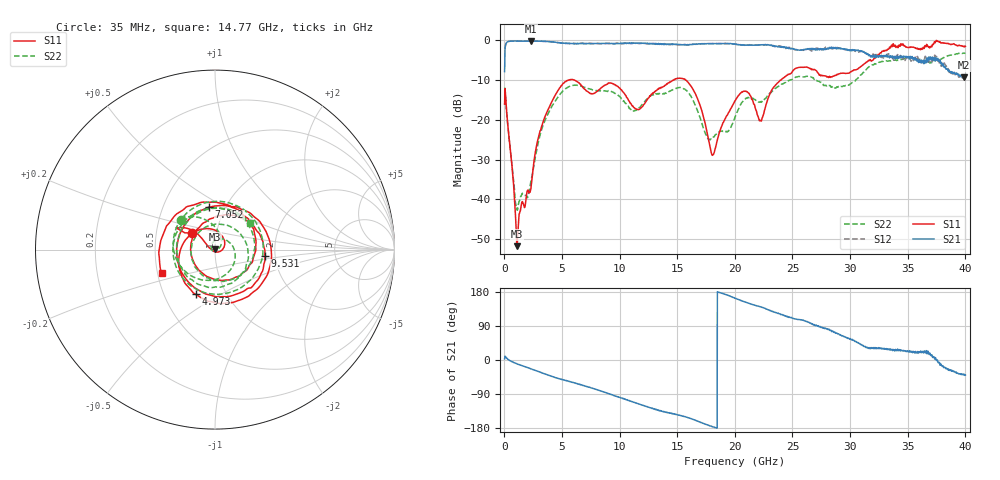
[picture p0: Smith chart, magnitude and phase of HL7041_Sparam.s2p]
! Created Wed Mar 30 16:31:27 2022
# ghz S ri R 50
! 2 Port Network Data from SP1.SP block
! freq  reS11  imS11  reS21  imS21  reS12  imS12  reS22  imS22
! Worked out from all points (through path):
!   2000 points, 35 MHz to 40 GHz, reference 50 ohm
!   highest |S21| = -0.13 dB at 2.354 GHz (marker M1); lowest = -9.3 dB at 39.86 GHz (marker M2)
!   group delay of S21, straight-line fit = 27.5 ps
!   lowest |S11| = -51.8 dB at 1.095 GHz (marker M3), VSWR 1.01, Z = 49.8 + j0.173 ohm
!   |S11| at or under -10 dB: start of sweep to 5.543 GHz; 6.107 GHz to 14.67 GHz (8.559 GHz wide, 82.4 % of centre); 15.75 GHz to 23.95 GHz (8.199 GHz wide, 41.3 % of centre)
!   |S22| runs from -42.7 to -3.2 dB; largest |S21 - S12| = 0.4
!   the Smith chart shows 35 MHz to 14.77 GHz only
!   S11 on the Smith chart (normalised r, x): 35 MHz: 0.76, +0.14; 4.973 GHz: 0.72, -0.39; 7.052 GHz: 0.84, +0.42; 9.531 GHz: 1.76, -0.14; 14.77 GHz: 0.53, -0.15
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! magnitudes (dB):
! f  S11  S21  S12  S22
! 35 MHz  -16.0  -7.8  -1.9  -12.1
! 1.095 GHz  -51.8  -0.1  -0.1  -42.2
! 2.354 GHz  -36.3  -0.1  -0.1  -35.0
! 3.214 GHz  -22.0  -0.2  -0.2  -22.7
! 4.973 GHz  -11.3  -0.7  -0.7  -13.1
! 6.712 GHz  -11.4  -0.8  -0.7  -11.6
! 7.052 GHz  -12.4  -0.8  -0.8  -11.9
! 9.531 GHz  -11.1  -0.8  -0.8  -13.2
! 11.57 GHz  -17.4  -0.7  -0.7  -17.3
! 13.37 GHz  -12.3  -0.8  -0.9  -13.5
! 14.77 GHz  -9.8  -1.0  -0.9  -12.2
! 16.47 GHz  -12.8  -1.0  -0.9  -15.6
! 18.07 GHz  -28.9  -0.8  -0.8  -24.7
! 20.03 GHz  -15.2  -0.9  -0.9  -19.2
! 21.09 GHz  -12.9  -1.2  -1.1  -14.4
! 22.25 GHz  -20.2  -1.1  -1.1  -15.4
! 23.73 GHz  -10.7  -1.6  -1.4  -11.6
! 26.68 GHz  -7.3  -2.2  -2.6  -9.2
! 29.7 GHz  -8.3  -2.3  -2.3  -11.4
! 33.34 GHz  -2.2  -3.9  -3.4  -5.1
! 39.86 GHz  -1.5  -9.3  -9.4  -3.2
! 40 GHz  -1.5  -9.1  -9.5  -3.2
